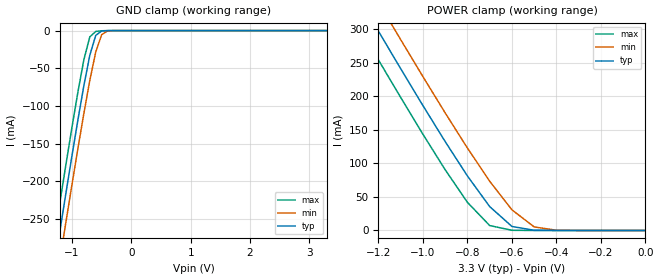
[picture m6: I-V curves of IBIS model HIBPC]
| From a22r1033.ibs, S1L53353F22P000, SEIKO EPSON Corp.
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[Model]   HIBPC
Model_type   Input
Polarity   Non-Inverting
Vinh=2.0V
Vinl=0.8V
|   typ   min   max
C_comp   5.0pF   4.0pF   6.0pF
|   typ   min   max
[Voltage range]   3.3   3.0   3.6
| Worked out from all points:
|   GND clamp passes 1 mA (typ) near -0.51 V on its own axis
|   POWER clamp passes 1 mA (typ) near -0.51 V on its own axis
[GND_clamp]
|   Voltage   I(typ)   I(min)   I(max)
-3.3V     -1.343A    -1.379A    -1.309A
-1.3V     -314.1mA   -352.4mA   -276.2mA
-1.2V     -264.1mA   -302.5mA   -226.1mA
-1.1V     -214.6mA   -253.1mA   -176.6mA
-1V       -165.9mA   -204.2mA   -128.1mA
-900mV    -118.4mA   -156.3mA   -81.33mA
-800mV    -73.08mA   -109.9mA   -38.6mA
-700mV    -32.75mA   -66.18mA   -8.318mA
-600mV    -6.318mA   -28.41mA   -1.129mA
-500mV    -586.9uA   -5.399mA   -239.5uA
-400mV    -56.77uA   -404.4uA   -18.72uA
3.3V      7.178nA    15.7uA     6.022nA
[POWER_clamp]
|   Voltage   I(typ)   I(min)   I(max)
-3.3V     1.514A     1.553A     1.476A
-1.3V     353.1mA    396.1mA    310.4mA
-1.2V     296.7mA    339.9mA    253.9mA
-1.1V     240.9mA    284.1mA    198mA
-1V       185.9mA    229mA      143.2mA
-900mV    132.3mA    175mA      90.33mA
-800mV    81.11mA    122.6mA    41.82mA
-700mV    35.52mA    73.27mA    7.314mA
-600mV    5.969mA    30.7mA     281.7uA
-500mV    284.1uA    5.285mA    30.01uA
-400mV    15.7uA     326.5uA    2.385uA
0V        7.178nA    15.84nA    7.223nA
